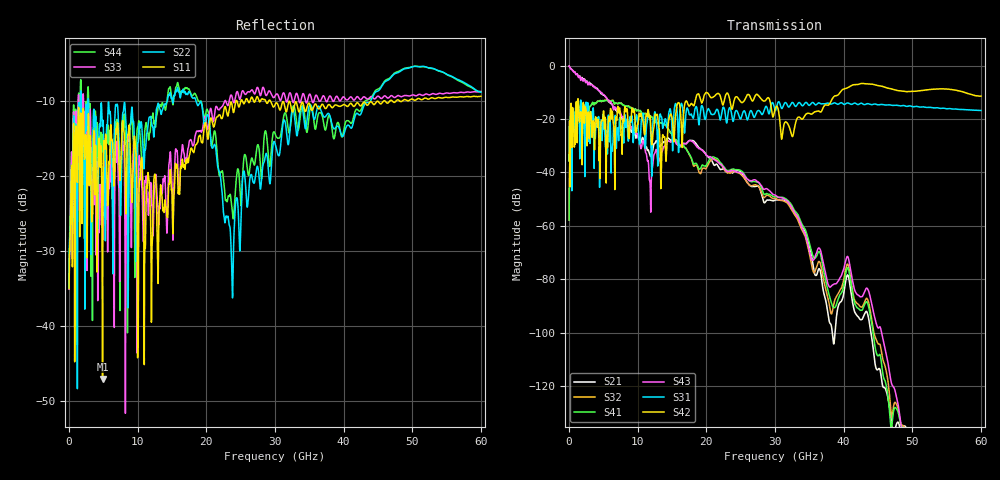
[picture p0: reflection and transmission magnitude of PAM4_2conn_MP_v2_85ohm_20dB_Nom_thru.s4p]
! Info: Touchstone file created by Circ.  Input file=FAB50GbE_2conn_Midplane_Examax_Topo2_v2_85ohm_20dB_Nom.circ
# Hz S RI R 50
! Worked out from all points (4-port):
!   6000 points, 10 MHz to 60 GHz, reference 50 ohm
!   strongest paths, dB at 10 MHz, 15.01 GHz, 30.01 GHz, 45.01 GHz, 60 GHz:
!     S42: -35.6, -19.6, -16.3, -7.5, -11.4
!     S31: -35.6, -24.7, -16.6, -14.7, -16.8
!     S43: -0.2, -27.9, -48.4, -98.2, -159.8
!     S41: -57.8, -26.0, -49.1, -108.7, -161.5
!     S32: -57.8, -26.1, -49.6, -104.1, -153.2
!     S21: -0.2, -27.9, -50.3, -113.8, -151.0
!   lowest |S11| = -47.0 dB at 4.88 GHz (marker M1), VSWR 1.01, Z = 50.3 - j0.296 ohm
!   |S11| at or under -10 dB: start of sweep to 24.31 GHz; 29.33 GHz to 45.85 GHz (16.51 GHz wide, 43.9 % of centre); 46 GHz to 46.75 GHz (749 MHz wide, 1.62 % of centre)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
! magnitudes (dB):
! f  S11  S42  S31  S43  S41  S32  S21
! 10 MHz  -35.0  -35.6  -35.6  -0.2  -57.8  -57.8  -0.2
! 1.06 GHz  -13.8  -13.4  -13.9  -3.4  -18.7  -18.9  -3.2
! 4.88 GHz  -47.0  -20.5  -21.4  -10.6  -13.1  -13.1  -10.7
! 11.87 GHz  -25.5  -21.1  -23.0  -51.2  -18.9  -19.0  -34.0
! 17.85 GHz  -16.3  -14.2  -18.4  -28.2  -34.7  -35.0  -28.0
! 37.07 GHz  -10.6  -15.5  -14.2  -74.2  -76.6  -80.1  -84.7
! 60 GHz  -9.4  -11.4  -16.8  -159.8  -161.5  -153.2  -151.0
